TYPE STR_Axis_Panasonic :
STRUCT
	Receive_Controlword_6040_00						:UINT;
	Receive_Modes_of_operation_6060_00				:SINT;
	Receive_Target_position_607A_00					:DINT;
	Receive_Touch_probe_function_60B8_00			:UINT;
	Receive_Home_offset_607C_00						:DINT;
	Receive_Speed_during_search_for_swi_6099_01		:UDINT;
	Receive_Speed_during_search_for_zer_6099_02		:UDINT;
	Receive_Homing_acceleration_609A_00				:UDINT;
	Receive_Homing_method_6098_00					:SINT;
	Transmit_Error_code_603F_00						:UINT;
	Transmit_Statusword_6041_00						:UINT;
	Transmit_Modes_of_operation_display_6061_00		:SINT;
	Transmit_Position_actual_value_6064_00			:DINT;
	Transmit_Velocity_actual_value_606C_00			:DINT;
	Transmit_Torque_actual_value_6077_00			:INT;
	Transmit_Touch_probe_status_60B9_00				:UINT;
	Transmit_Touch_probe_pos1_pos_value_60BA_00		:DINT;
	Transmit_Touch_probe_pos1_neg_value_60BB_00		:DINT;
	Transmit_Digital_inputs_60FD_00					:UDINT;
END_STRUCT
END_TYPE
